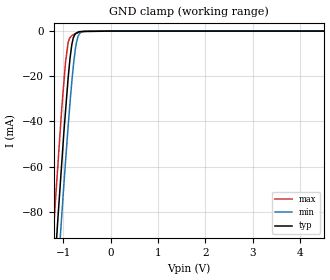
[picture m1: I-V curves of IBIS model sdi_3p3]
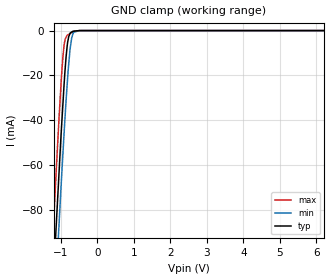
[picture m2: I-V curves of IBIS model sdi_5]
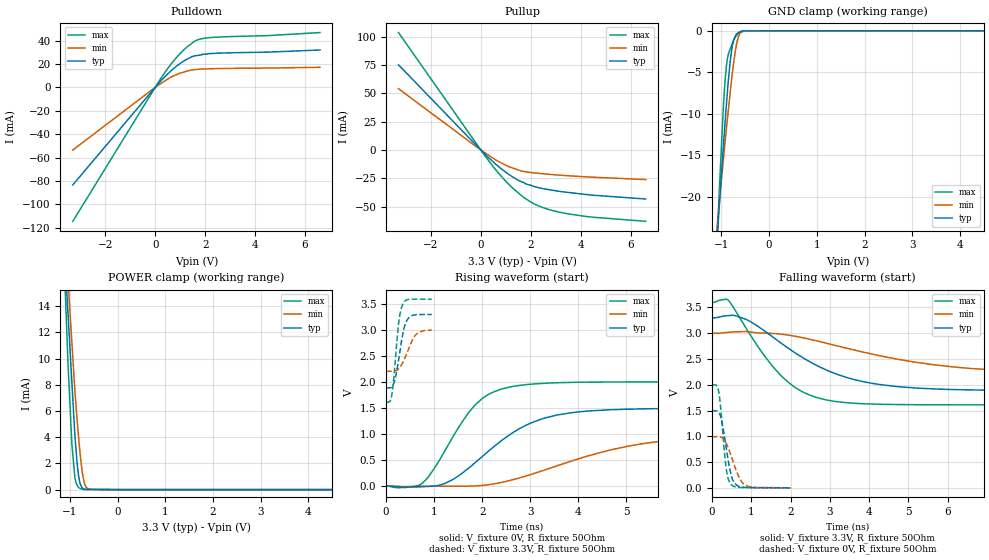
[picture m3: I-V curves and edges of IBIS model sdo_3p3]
|Texas Instruments Incorporated
| 16-bit, Unipolar differential input, 500kSPS Serial Out,
|  4.5V to 5.5V Micro Power Sampling ADC
| Marketing part#   Digital Voltage Range   Package-type   #pins
| ADS8318IBDGSR   2.375 to 5.5V   MSOP   10
| ADS8318IBDGSRG4   2.375 to 5.5V   MSOP   10
| ADS8318IBDGST   2.375 to 5.5V   MSOP   10
| ADS8318IBDGSTG4   2.375 to 5.5V   MSOP   10
| ADS8318IBDRCR   2.375 to 5.5V   SON   10
| ADS8318IBDRCRG4   2.375 to 5.5V   SON   10
| ADS8318IBDRCT   2.375 to 5.5V   SON   10
| ADS8318IBDRCTG4   2.375 to 5.5V   SON   10
| ADS8318IDGSR   2.375 to 5.5V   MSOP   10
| ADS8318IDGSRG4   2.375 to 5.5V   MSOP   10
| ADS8318IDGST   2.375 to 5.5V   MSOP   10
| ADS8318IDGSTG4   2.375 to 5.5V   MSOP   10
| ADS8318IDRCR   2.375 to 5.5V   SON   10
| ADS8318IDRCRG4   2.375 to 5.5V   SON   10
| ADS8318IDRCT   2.375 to 5.5V   SON   10
| ADS8318IDRCTG4   2.375 to 5.5V   SON   10
[IBIS Ver]   3.2
[File name]   ads8318.ibs
|SIMDE Ver   V2.2 - 201009 - RHL4 - Build 420
[File Rev]   1.0
[Date]   12/8/2010
[Source]
| Texas Instruments Incorporated.
| Analog-eLab Design Center, HPA
| 12500 TI Blvd
| Dallas, TX -75243
| e-mail: elab_ibis@list.ti.com
| -Model generated from simulations in TISPICE
[Notes]   Revision History:
| Rev 1.0: 12/8/2010
| - Initial version of the model
| - Model generated from simulations in TISPICE
| - Model matched to SPICE simulation
| - Model names with a trailing 3p3 contains the model for
|   3.3V [3.0V and 3.6V]. Model names with trailing 5 contains
|   the model for 5.0V [4.5V and 5.5V] operation.
| - C_comp although listed in numerical order of value are
|   obtained from varying PVT conditions. For PVT conditions for
|   each specific value refer the buffer description under
|   respective [Model]. IBIS model user is responsible for using
|   appropriate C_comp to simulate for Signal Integrity.
[Disclaimer]
| This model is designed as an aid for customers of Texas Instruments.
| TI and its licensors and suppliers make no warranties, either expressed
| or implied, with respect to this  model, including the warranties of
| merchantability or fitness for a particular purpose. The model is
| provided solely on an "as is" basis. The entire risk as to its quality
| and performance is with the customer.
[Copyright]
 (C) Copyright 2010 Texas Instruments Incorporated.All rights reserved.
|   ADS8318DRC
[Component]   ADS8318DRC
[Manufacturer]   TI
[Package]   |10 SON  -  DRC package
|   typ   min   max
R_pkg   0.04535   0.04466   0.04641
L_pkg   0.81550nH   0.75877nH   0.88863nH
C_pkg   0.21288pF   0.16197pF   0.27626pF
[Pin]  signal_name   model_name   R_pin   L_pin   C_pin
1   REFIN   TERM   0.04609   0.88643nH  0.23102pF
2   +VA   POWER   0.04639   0.88452nH  0.26571pF
3   IN+   TERM   0.04621   0.88428nH  0.26086pF
4   IN-   TERM   0.04641   0.88863nH  0.27626pF
5   GND   GND   0.02313   0.57163nH  0.27592pF
6   CONVST   SDI   0.04476   0.77072nH  0.16197pF
7   SDO   SDO   0.04466   0.75981nH  0.18663pF
8   SCLK   SDI   0.04466   0.75877nH  0.18676pF
9   SDI   SDI   0.04467   0.75987nH  0.18669pF
10   +VBD   POWER   0.04468   0.76955nH  0.16191pF
|   ADS8318DGS
[Component]   ADS8318DGS
[Manufacturer]   TI
[Package]   |10 MSOP -  DGS package
|   typ   min   max
R_pkg   0.03477   0.03469   0.03498
L_pkg   0.58765nH   0.56717nH   0.61794nH
C_pkg   0.16612pF   0.14840pF   0.17988pF
[Pin]  signal_name   model_name   R_pin   L_pin   C_pin
1   REFIN   TERM   0.03482   0.61794nH  0.15473pF
2   +VA   POWER   0.03502   0.61579nH  0.16915pF
3   IN+   TERM   0.03477   0.60993nH  0.16899pF
4   IN-   TERM   0.03498   0.60766nH  0.17988pF
5   GND   GND   0.01811   0.41560nH  0.20604pF
6   CONVST   SDI   0.03469   0.57469nH  0.14840pF
7   SDO   SDO   0.03474   0.56840nH  0.17024pF
8   SCLK   SDI   0.03471   0.56717nH  0.17035pF
9   SDI   SDI   0.03470   0.56777nH  0.17024pF
10   +VBD   POWER   0.03469   0.57469nH  0.14846pF
|   Model Selectors
[Model Selector] SDI
sdi_3p3   3.3V digital input
sdi_5   5.0V digital input
[Model Selector] SDO
sdo_3p3   3.3V digital output
sdo_5   5.0V digital output
[Model Selector] TERM
term_3-3V  3.3V nominal termination
term_5-0V  5.0V nominal termination
[Model]  term_3-3V
Model_type Terminator
C_comp   1.0e-20F  1.0e-20F  1.0e-20F
|   typ   min   max
[Voltage Range]   3.3V   3.0V   3.6V
[POWER Clamp Reference]   3.3V   3.0V   3.6V
[GND Clamp Reference]   0V   0V   0V
|Ambient Temperature   25   85   -40
|Junction Temperature
[Temperature Range]   28   89   -40
[Model]  term_5-0V
Model_type Terminator
C_comp   1.0e-20F  1.0e-20F  1.0e-20F
|   typ   min   max
[Voltage Range]   5.0V   4.5V   5.5V
[POWER Clamp Reference]   5.0V   4.5V   5.5V
[GND Clamp Reference]   0V   0V   0V
|Ambient Temperature   25   85   -40
|Junction Temperature
[Temperature Range]   28   89   -40
| Models and submodels in the file (6): sdi_3p3 (Input), sdi_5 (Input), sdo_3p3 (3-state), sdo_5 (3-state), term_3-3V (Terminator), term_5-0V (Terminator)
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|   sdi_3p3 Model
[Model]   sdi_3p3
Model_type   Input
Vinl = 1.08
Vinh = 2.1
|   typ   min   max
|   (Nom PVT)   (Fast PVT)   (Slow PVT)
|C_comp from frequency method
|Average
|C_comp   9.887e-13   1.119e-12   8.638e-13
|C_comp from L-C Tank method
|Average
C_comp   7.41E-13   6.92E-13   8.01E-13
| Where nom  PVT is Nominal Process,  3.3V,  28C
|   Fast PVT is Strong Process,   3.6V,  -40C
|   Slow PVT is Weak Process,   3V,  89C
[Model Spec]
Vinl   0.99   0.9   1.08
Vinh   2.31   2.1   2.52
[Voltage Range]   3.3   3   3.6
|Ambient Temperature   25   85   -40
|Junction Temperature
[Temperature Range]   28   89   -40
[Power Clamp Reference]   3.3   3   3.6
[GND Clamp Reference]   0   0   0
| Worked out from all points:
|   GND clamp passes 1 mA (typ) near -0.73 V on its own axis
[GND Clamp]
|   Voltage   I(typ)   I(min)   I(max)
-3.3V     -824mA     -839.5mA   -807mA
-1.29V    -139.6mA   -163.5mA   -115.9mA
-1.166V   -99.85mA   -123.2mA   -75.3mA
-1.143V   -92.34mA   -115.7mA   -68.11mA
-1.115V   -83.48mA   -107.2mA   -59.63mA
-1.037V   -59.68mA   -82.95mA   -35.47mA
-954mV    -35.8mA    -58.11mA   -13.96mA
-896.4mV  -20.47mA   -41.86mA   -4.929mA
-788.7mV  -2.985mA   -15.73mA   -1.6mA
-741mV    -1.102mA   -7.411mA   -1.124mA
-673.2mV  -326.4uA   -1.703mA   -480.6uA
6.6V      0A         0A         0A
[POWER Clamp]
|   Voltage   I(typ)   I(min)   I(max)
-3.3V     0A         0A         0A
6.6V      0A         0A         0A
|   sdi_5 Model
[Model]   sdi_5
Model_type   Input
Vinl = 1.65
Vinh = 3.15
|   typ   min   max
|   (Nom PVT)   (Fast PVT)   (Slow PVT)
|C_comp from frequency method
|Average
|C_comp   9.396e-13   1.057e-12   8.279e-13
|C_comp from L-C Tank method
|Average
C_comp   7.24E-13   6.79E-13   7.76E-13
| Where nom  PVT is Nominal Process,  5V,  28C
|   Fast PVT is Strong Process,   5.5V,  -40C
|   Slow PVT is Weak Process,   4.5V,  89C
[Model Spec]
Vinl   1.5   1.35   1.65
Vinh   3.5   3.15   3.85
[Voltage Range]   5   4.5   5.5
|Ambient Temperature   25   85   -40
|Junction Temperature
[Temperature Range]   28   89   -40
[Power Clamp Reference]   5   4.5   5.5
[GND Clamp Reference]   0   0   0
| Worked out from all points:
|   GND clamp passes 1 mA (typ) near -0.74 V on its own axis
[GND Clamp]
|   Voltage   I(typ)   I(min)   I(max)
-5V       -1.411A    -1.423A    -1.399A
-1.368V   -165.2mA   -188mA     -141.5mA
-1.202V   -111.2mA   -134.2mA   -87.08mA
-1.133V   -89.09mA   -112.7mA   -64.7mA
-1.062V   -67.44mA   -90.46mA   -42.98mA
-946mV    -33.6mA    -55.85mA   -12.29mA
-907.5mV  -23.2mA    -44.96mA   -6.071mA
-855mV    -11.56mA   -30.92mA   -2.939mA
-815mV    -5.412mA   -21.47mA   -1.968mA
-751.5mV  -1.468mA   -8.939mA   -1.354mA
-670mV    -309.6uA   -1.485mA   -564.3uA
10V       0A         0A         0A
[POWER Clamp]
|   Voltage   I(typ)   I(min)   I(max)
-5V       0A         0A         0A
10V       0A         0A         0A
|   sdo_3p3 Model
[Model]   sdo_3p3
Model_type   3-state
Polarity   Inverting
Enable   Active-High
Vmeas = 1.65
Vref = 1.65
Cref = 5pF
Rref = 50
|   typ   min   max
|   (Nom PVT)   (Fast PVT)   (Slow PVT)
|C_comp from frequency method
|Average
|C_comp   3.368e-12   2.896e-12   4.009e-12
|ON state : BUFFER OUTPUT TURNED HIGH
|C_comp   3.368e-12   2.896e-12   4.009e-12
|OFF state: BUFFER IN HIGH IMPEDANCE
|C_comp   1.245e-12   1.046e-12   1.452e-12
|C_comp from LC tank method
C_comp   1.157e-12   9.649e-13   1.366e-12
| Where nom  PVT is Nominal Process,  3.3V,  28C
|   Fast PVT is Strong Process,   3.6V,  -40C
|   Slow PVT is Weak Process,   3V,  89C
[Voltage Range]   3.3   3   3.6
|Ambient Temperature   25   85   -40
|Junction Temperature
[Temperature Range]   28   89   -40
[Pullup Reference]   3.3   3   3.6
[Pulldown Reference]   0   0   0
[Power Clamp Reference]   3.3   3   3.6
[GND Clamp Reference]   0   0   0
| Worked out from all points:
|   slope of the pulldown table from 0 to 0.495 V, typ, clamps not added: 43.8 ohm
|   slope of the pullup table from 0 to 0.495 V, typ, clamps not added: 47.5 ohm
|   GND clamp passes 1 mA (typ) near -0.74 V on its own axis
|   POWER clamp passes 1 mA (typ) near -0.82 V on its own axis
|   falling waveform, V_fixture 3.3V, R_fixture 50Ohm: 20-80 % time 1.94ns typ, 3.18ns min, 1.22ns max; typ from 3.3 V to 1.89 V
|   rising waveform, V_fixture 0V, R_fixture 50Ohm: 20-80 % time 1.32ns typ, 2.27ns min, 859ps max; typ from 0 V to 1.49 V
|   rising waveform, V_fixture 3.3V, R_fixture 50Ohm: 20-80 % time 155ps typ, 224ps min, 117ps max; typ from 1.89 V to 3.29 V
|   falling waveform, V_fixture 0V, R_fixture 50Ohm: 20-80 % time 197ps typ, 290ps min, 142ps max; typ from 1.49 V to 0.002 V
[Pulldown]
|   Voltage   I(typ)   I(min)   I(max)
-3.3V     -83.41mA   -53.59mA   -114.5mA
172.8mV   4.268mA    2.468mA    5.912mA
478.8mV   10.98mA    6.77mA     15.47mA
738mV     16.09mA    9.845mA    22.63mA
1.246V    23.77mA    13.66mA    34.04mA
1.573V    26.88mA    15.14mA    39.33mA
1.818V    27.69mA    15.57mA    41.44mA
2.012V    28.33mA    15.74mA    42.16mA
2.627V    29.3mA     16.09mA    43.06mA
4.5V      30.11mA    16.48mA    44.22mA
6.6V      31.95mA    17.16mA    46.85mA
[GND Clamp]
|   Voltage   I(typ)   I(min)   I(max)
-3.3V     -235.4mA   -169.8mA   -358.6mA
-1.129V   -28.49mA   -25.99mA   -30.79mA
-1.044V   -21.1mA    -20.7mA    -19.22mA
-957.6mV  -13.84mA   -15.44mA   -9.034mA
-925.2mV  -11.24mA   -13.53mA   -6.121mA
-896.4mV  -8.941mA   -11.84mA   -4.274mA
-849.6mV  -5.704mA   -9.295mA   -2.7mA
-782.1mV  -2.173mA   -5.645mA   -1.681mA
-742.5mV  -1.068mA   -3.806mA   -1.152mA
-699mV    -529.2uA   -2.11mA    -692.2uA
-603.9mV  -76.01uA   -256.6uA   -198.7uA
6.6V      0A         0A         0A
[Pullup]
|   Voltage   I(typ)   I(min)   I(max)
-3.3V     75.19mA    54.14mA    103.6mA
18mV      -398.8uA   -290.5uA   -564.7uA
478.8mV   -10.1mA    -7.041mA   -14.21mA
939.6mV   -18.58mA   -12.67mA   -26.15mA
1.202V    -22.65mA   -15.22mA   -32.1mA
1.706V    -28.54mA   -18.8mA    -41.6mA
1.806V    -29.88mA   -19.15mA   -43.07mA
2.2V      -32.58mA   -20.23mA   -48.16mA
2.473V    -33.89mA   -20.87mA   -50.65mA
3.089V    -36.21mA   -21.98mA   -54.5mA
4.496V    -39.8mA    -23.92mA   -59.21mA
6.6V      -43.12mA   -26.03mA   -62.79mA
[POWER Clamp]
|   Voltage   I(typ)   I(min)   I(max)
-3.3V     146mA      129.1mA    169.7mA
-1.096V   16.91mA    19.21mA    14.82mA
-1.037V   13.12mA    15.74mA    9.229mA
-961.2mV  8.255mA    11.29mA    3.519mA
-896.4mV  4.103mA    7.486mA    876.6uA
-858mV    2.327mA    5.659mA    398.2uA
-818.4mV  1.026mA    3.93mA     166.1uA
-774mV    349.3uA    2.26mA     56.03uA
-741mV    116.4uA    1.301mA    35.05uA
-693mV    23.58uA    442.2uA    5.634uA
-591mV    20.09uA    22.11uA    3.37uA
6.6V      0A         0A         0A
[Ramp]
R_load = 50
|   typ   min   max
dV/dt_r   0.896331/1.32013e-09   0.595401/2.27723e-09   1.19939/8.54006e-10
dV/dt_f   0.849069/1.93379e-09   0.475443/3.17421e-09   1.19342/1.22272e-09
[Falling Waveform]
V_fixture = 3.3V
V_fixture_min = 3V
V_fixture_max = 3.6V
R_fixture = 50Ohm
|   Time   V(typ)   V(min)   V(max)
0s        3.3V       3V         3.6V
415ps     3.341V     3.017V     3.642V
905ps     3.255V     3.033V     3.055V
1.295ns   3.068V     3.003V     2.606V
1.745ns   2.817V     2.983V     2.189V
2.28ns    2.541V     2.917V     1.874V
2.915ns   2.285V     2.806V     1.706V
4.295ns   2.002V     2.559V     1.622V
6.595ns   1.9V       2.316V     1.611V
12.99ns   1.885V     2.208V     1.611V
[Rising Waveform]
V_fixture = 0V
V_fixture_min = 0V
V_fixture_max = 0V
R_fixture = 50Ohm
|   Time   V(typ)   V(min)   V(max)
0s        1.015nV    1.177nV    912pV
750ps     -4.564mV   -15.03mV   53.38mV
1.235ns   54.06mV    -2.251mV   697.4mV
1.85ns    447.7mV    2.535mV    1.553V
2.155ns   690.1mV    28.92mV    1.772V
2.605ns   1.005V     113.2mV    1.907V
3.56ns    1.364V     389.2mV    1.983V
4.67ns    1.464V     692.9mV    1.997V
5.755ns   1.487V     865.3mV    1.999V
9.87ns    1.494V     988.9mV    1.999V
[Rising Waveform]
V_fixture = 3.3V
V_fixture_min = 3V
V_fixture_max = 3.6V
R_fixture = 50Ohm
|   Time   V(typ)   V(min)   V(max)
0s        1.885V     2.205V     1.611V
74.35ps   1.884V     2.205V     1.622V
114.6ps   1.898V     2.203V     1.735V
186.9ps   2.062V     2.208V     2.368V
259.2ps   2.419V     2.25V      3.119V
340.2ps   2.893V     2.36V      3.48V
412.6ps   3.143V     2.506V     3.567V
487.9ps   3.245V     2.679V     3.586V
630.9ps   3.288V     2.918V     3.587V
948.9ps   3.292V     2.995V     3.586V
[Falling Waveform]
V_fixture = 0V
V_fixture_min = 0V
V_fixture_max = 0V
R_fixture = 50Ohm
|   Time   V(typ)   V(min)   V(max)
0s        1.492V     992.3mV    1.995V
116.1ps   1.495V     994.7mV    1.989V
178.4ps   1.463V     996.6mV    1.852V
251.2ps   1.3V       979.5mV    1.322V
355.3ps   827.7mV    879mV      432.9mV
407.8ps   568.9mV    790.7mV    199.1mV
470.9ps   312mV      661.7mV    81.48mV
603.6ps   70.27mV    369.9mV    19.53mV
838.6ps   11.65mV    57.76mV    5.484mV
2ns       2.058mV    2.862mV    1.412mV
